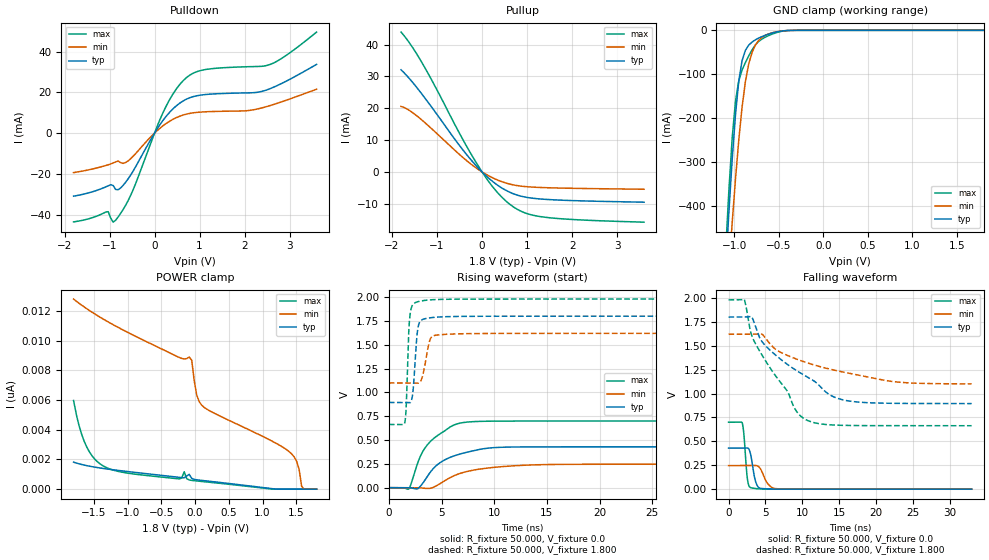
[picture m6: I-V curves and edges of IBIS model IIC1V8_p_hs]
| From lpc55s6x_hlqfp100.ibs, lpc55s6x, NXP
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|   Model IIC1V8_p_hs
[Model] IIC1V8_p_hs
Model_type I/O
Polarity   Non-Inverting
Enable   Active-Low
Vinl =  0.540V
Vinh =  1.260V
Vmeas =  0.900V
Cref =  0.0F
Rref =  100.000
Vref =  0.0V
C_comp   2.515pF   2.512pF   2.535pF
C_comp_pullup   0.454pF   0.388pF   0.548pF
C_comp_pulldown   1.734pF   1.669pF   1.790pF
[Model Spec]
Vinh   1.260V   1.134V   1.386V
Vinl   0.540V   0.486V   0.594V
Vmeas   0.900V   0.810V   0.990V
Vref   0.0V   0.0V   0.0V
Cref   0.0F   0.0F   0.0F
Rref   1000.000   1000.000   1000.000
[Temperature Range]   25.000   0.125k   -40.000
[Voltage Range]   1.800V   1.620V   1.980V
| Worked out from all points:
|   slope of the pulldown table from 0 to 0.27 V, typ, clamps not added: 31.5 ohm
|   slope of the pullup table from 0 to 0.27 V, typ, clamps not added: 79.6 ohm
|   GND clamp passes 1 mA (typ) near -0.44 V on its own axis
|   rising waveform, R_fixture 50.000, V_fixture 0.0: 20-80 % time 2.98ns typ, 3.78ns min, 2.4ns max; typ from 0 V to 0.429 V
|   rising waveform, R_fixture 50.000, V_fixture 1.800: 20-80 % time 347ps typ, 537ps min, 255ps max; typ from 0.894 V to 1.8 V
|   falling waveform, R_fixture 50.000, V_fixture 0.0: 20-80 % time 599ps typ, 965ps min, 409ps max; typ from 0.429 V to 0 V
|   falling waveform, R_fixture 50.000, V_fixture 1.800: 20-80 % time 8.38ns typ, 11.2ns min, 5.71ns max; typ from 1.8 V to 0.895 V
[Pulldown]
|Voltage   I(typ)   I(min)   I(max)
-1.8V     -30.97mA   -19.41mA   -43.61mA
-1.03V    -25.91mA   -15.56mA   -38.59mA
-920mV    -25.75mA   -14.67mA   -43.75mA
-865mV    -27.69mA   -14.16mA   -42.79mA
-700mV    -25.69mA   -14.87mA   -37.58mA
-480mV    -18.8mA    -11.48mA   -28.03mA
235mV     7.619mA    4.356mA    12.23mA
455mV     12.83mA    7.267mA    20.76mA
730mV     16.88mA    9.427mA    27.6mA
1.17V     19mA       10.49mA    31.33mA
2.545V    21.62mA    13.37mA    33.53mA
3.6V      33.73mA    21.54mA    49.59mA
[Pullup]
|Voltage   I(typ)   I(min)   I(max)
-1.8V     32.07mA    20.56mA    43.91mA
-1.57V    28.57mA    18.88mA    39.63mA
-1.295V   23.66mA    15.78mA    33.32mA
-1.02V    18.41mA    12.25mA    26.23mA
-470mV    7.716mA    5.078mA    11.29mA
-30mV     432.2uA    271.3uA    660.2uA
300mV     -3.713mA   -2.28mA    -5.781mA
630mV     -6.475mA   -3.874mA   -10.31mA
960mV     -7.909mA   -4.606mA   -12.9mA
1.4V      -8.61mA    -4.943mA   -14.23mA
2.17V     -9.075mA   -5.188mA   -15.07mA
3.6V      -9.515mA   -5.442mA   -15.79mA
[GND_clamp]
|Voltage   I(typ)   I(min)   I(max)
-1.8V     -3.488A    -3.23A     -3.872A
-1.097V   -545.5mA   -658.5mA   -507mA
-1.06V    -414.6mA   -546.1mA   -365mA
-1.023V   -294.9mA   -439.1mA   -245.9mA
-986mV    -192.4mA   -339.5mA   -162mA
-949mV    -115.6mA   -250.3mA   -115.1mA
-912mV    -69.18mA   -175.2mA   -90.61mA
-838mV    -34.01mA   -77.15mA   -58.49mA
-764mV    -21.81mA   -34.1mA    -33.59mA
-653mV    -11.42mA   -11.64mA   -15.82mA
-431mV    -827.9uA   -873.5uA   -1.132mA
1.8V      0A         0A         0A
[POWER_clamp]
|Voltage   I(typ)   I(min)   I(max)
-1.8V     1.82nA     12.81nA    5.971nA
-1.604V   1.585nA    12.15nA    2.835nA
-1.271V   1.34nA     11.22nA    1.374nA
-161mV    762.4pA    8.77nA     1.175nA
-87mV     998.4pA    8.9nA      618.7pA
-50mV     731.2pA    8.692nA    590.6pA
24mV      632.5pA    6.343nA    553.1pA
98mV      590.6pA    5.66nA     518.6pA
1.356V    0A         2.658nA    0A
1.504V    0A         1.877nA    0A
1.578V    0A         193.2pA    0A
1.8V      0A         0A         0A
[Ramp]
| variable   typ   min   max
dV/dt_r   0.257/2.981n   0.148/3.782n   0.420/2.396n
dV/dt_f   0.543/8.378n   0.311/11.179n   0.790/5.713n
R_load = 50.000
[Rising Waveform]
R_fixture= 50.000
V_fixture= 0.0
V_fixture_min= 0.0
V_fixture_max= 0.0
|time   V(typ)   V(min)   V(max)
0s        7.217nV    72.68nV    5.104nV
1.899ns   195uV      -156.2nV   -12.48mV
2.768ns   -9.184mV   -27.26uV   269.8mV
3.581ns   106.1mV    -8.139mV   440.1mV
4.871ns   263.3mV    42.75mV    566mV
5.981ns   325.5mV    115.4mV    647.8mV
6.841ns   356.1mV    152.6mV    679.4mV
9.482ns   415.8mV    207.5mV    697.9mV
13.67ns   428.3mV    239.1mV    699.6mV
33ns      429mV      246.4mV    699.8mV
[Rising Waveform]
R_fixture= 50.000
V_fixture= 1.800
V_fixture_min= 1.620
V_fixture_max= 1.980
|time   V(typ)   V(min)   V(max)
0s        894.4mV    1.099V     663.4mV
1.516ns   894.4mV    1.099V     687.8mV
1.638ns   894.6mV    1.099V     838mV
1.974ns   891.8mV    1.099V     1.783V
2.282ns   1.006V     1.099V     1.923V
2.635ns   1.559V     1.097V     1.949V
2.994ns   1.749V     1.115V     1.958V
3.883ns   1.783V     1.547V     1.971V
4.436ns   1.789V     1.6V       1.975V
33ns      1.8V       1.62V      1.98V
[Falling Waveform]
R_fixture= 50.000
V_fixture= 0.0
V_fixture_min= 0.0
V_fixture_max= 0.0
|time   V(typ)   V(min)   V(max)
0s        429.1mV    246.5mV    699.9mV
1.864ns   429.1mV    246.5mV    691.6mV
2.084ns   429mV      246.5mV    573.3mV
2.567ns   430.6mV    246.5mV    103.4mV
3.083ns   330.7mV    246.5mV    13.81mV
3.705ns   71.99mV    247.6mV    5.792mV
4.495ns   7.249mV    189.6mV    2.214mV
5.381ns   2.677mV    51.99mV    923.1uV
6.461ns   1.069mV    5.305mV    378.2uV
33ns      1.301uV    2.937uV    622.3nV
[Falling Waveform]
R_fixture= 50.000
V_fixture= 1.800
V_fixture_min= 1.620
V_fixture_max= 1.980
|time   V(typ)   V(min)   V(max)
0s        1.8V       1.62V      1.98V
2.135ns   1.8V       1.62V      1.984V
2.917ns   1.806V     1.62V      1.668V
3.531ns   1.73V      1.62V      1.539V
5.101ns   1.493V     1.57V      1.332V
7.99ns    1.304V     1.398V     1.025V
9.234ns   1.24V      1.36V      813.2mV
10.51ns   1.182V     1.326V     726.7mV
16.18ns   923.9mV    1.215V     666.4mV
33ns      895mV      1.101V     663.5mV
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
